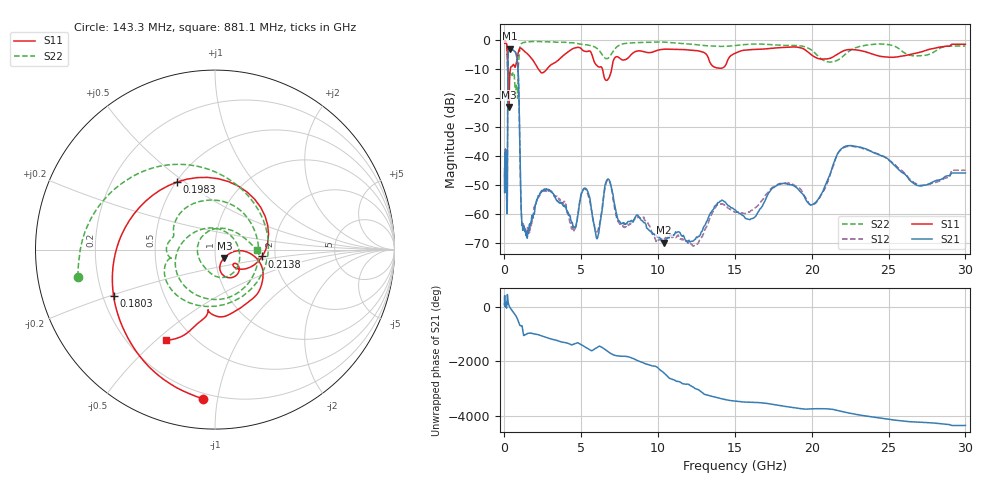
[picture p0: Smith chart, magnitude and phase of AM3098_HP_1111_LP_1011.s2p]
! Date/Time: Thu, Feb 28, 2019 8:48 AM
! Network Analyzer: Agilent Technologies E8364B Rev: A.07.50.67
! Sweep from 0.010 to 30.000 GHz, 1601 Points, Sweep Type: LOG
! Power Supply: 5.022 V, 0.002 A
# Hz S DB R 50
!freq MagS11 AngS11 MagS21 AngS21 MagS12 AngS12 MagS22 AngS22
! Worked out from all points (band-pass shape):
!   1601 points, 10 MHz to 30 GHz, reference 50 ohm
!   highest |S21| = -3.11 dB at 340.5 MHz (marker M1); lowest = -69.8 dB at 10.38 GHz (marker M2)
!   |S21| within 3 dB of the highest: 228.4 MHz to 807.4 MHz (578.9 MHz wide, 112 % of centre)
!   lowest |S11| = -23.2 dB at 293 MHz (marker M3), VSWR 1.15, Z = 55.2 - j5.13 ohm
!   |S11| at or under -10 dB: 210.1 MHz to 385 MHz (174.9 MHz wide, 58.8 % of centre); 2.196 GHz to 2.779 GHz (582.9 MHz wide, 23.4 % of centre); 6.372 GHz to 6.98 GHz (608.4 MHz wide, 9.11 % of centre)
!   |S22| runs from -20.1 to -0.6 dB; largest |S21 - S12| = 0.01
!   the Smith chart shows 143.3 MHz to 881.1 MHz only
!   S11 on the Smith chart (normalised r, x): 143.3 MHz: 0.17, -0.91; 180.3 MHz: 0.24, -0.20; 198.3 MHz: 0.51, +0.47; 213.8 MHz: 1.71, -0.14; 881.1 MHz: 0.36, -0.54
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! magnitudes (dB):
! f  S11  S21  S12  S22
! 10 MHz  -0.3  -44.2  -46.4  -0.6
! 38.04 MHz  -0.2  -40.7  -40.7  -0.7
! 97.46 MHz  -0.8  -38.9  -38.4  -1.5
! 143.3 MHz  -1.6  -51.9  -56.4  -2.2
! 144.7 MHz  -1.6  -52.5  -57.0  -2.2
! 180.3 MHz  -4.1  -56.1  -57.2  -5.3
! 198.3 MHz  -7.3  -36.8  -36.5  -10.5
! 213.8 MHz  -11.5  -12.8  -12.8  -9.6
! 293 MHz  -23.2  -3.3  -3.2  -12.2
! 340.5 MHz  -12.7  -3.1  -3.1  -11.6
! 550.5 MHz  -8.7  -3.6  -3.5  -11.3
! 881.1 MHz  -4.8  -10.1  -10.0  -12.6
! 1.16 GHz  -3.2  -63.4  -63.8  -1.1
! 2.084 GHz  -9.0  -55.6  -55.5  -0.6
! 5.258 GHz  -4.0  -51.1  -51.3  -1.7
! 6.019 GHz  -8.9  -68.4  -66.1  -2.9
! 6.753 GHz  -13.5  -47.9  -48.0  -6.3
! 7.926 GHz  -6.7  -63.1  -64.2  -1.2
! 10.38 GHz  -3.2  -69.8  -68.8  -0.8
! 20.1 GHz  -5.6  -56.5  -56.8  -4.1
! 22.56 GHz  -3.4  -36.4  -36.5  -3.5
! 30 GHz  -1.5  -45.8  -44.9  -2.2
